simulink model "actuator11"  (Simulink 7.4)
settings: Solver=ode45  StartTime=0.0  StopTime=.35  MaxStep=1e-4  RelTol=1e-3
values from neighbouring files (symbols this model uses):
  D = str2num(get(h,'string'))    [acttrcalc1.m]
  fa = str2num(get(h,'string'))    [actsscalc1.m]    (also in acttrcalc1.m; calc0.m = f)
  k = str2num(get(h,'string'))    [actsscalc1.m]    (also in acttrcalc1.m; dcm.m = menu('DC MACHINES DEMOS:','DC motor transient running operat; dtcvectorselection.m = 1:6; dtcvectorsmovie.m = 1:6)
  K = 2.5    [actss.m]    (also in actsscalc1.m = str2num(get(h,'string')); acttrcalc1.m = str2num(get(h,'string')))
  M = length(wmm)    [Actac.m]    (also in acttrcalc1.m = str2num(get(h,'string')); calc0.m = fix(tf/ti))
  R = str2num(get(h,'string'))    [acttrcalc1.m]    (also in IMabc2.m = diag([Rs Rs Rs Rr Rr Rr]); IMabcf0.m = diag([Rs Rs Rs Rr Rr Rr]); IMabcf1.m = diag([Rs Rs Rs Rr Rr Rr]); IMcurf0.m = diag([Rs Rs Rr Rr]))
  V = [Vas 0 0].'    [Actac.m]    (also in acttrcalc1.m = str2num(get(h,'string')); im3d.m = eval(get(hVs,'String')); IMabc2.m = [vas vbs vcs 0 0 0]'; IMabcf0.m = [vas vbs vcs 0 0 0]')
  xsi = str2num(get(h,'string'))    [actsscalc1.m]    (also in acttrcalc1.m)

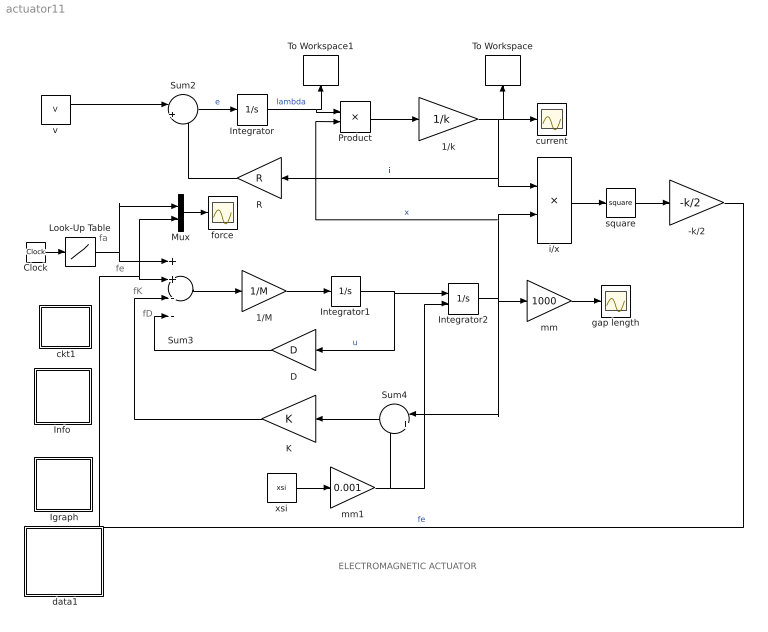
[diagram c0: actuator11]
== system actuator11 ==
  note: ELECTROMAGNETIC ACTUATOR
  note: fe
  note: fa
  note: fK
  note: fD
  " Igraph" : Subsystem
  " ckt1" : Subsystem
  " data1" : Subsystem
  -k/2 : Gain  Gain=-k/2  ParameterDataType=sfix(16)  ParameterScaling=2^0  OutDataType=sfix(16)  OutScaling=2^0
  1/M : Gain  Gain=1/M  ParameterDataType=sfix(16)  ParameterScaling=2^0  OutDataType=sfix(16)  OutScaling=2^0
  1/k : Gain  Gain=1/k  ParameterDataType=sfix(16)  ParameterScaling=2^0  OutDataType=sfix(16)  OutScaling=2^0
  Clock : Clock
  D : Gain  Gain=D  ParameterDataType=sfix(16)  ParameterScaling=2^0  OutDataType=sfix(16)  OutScaling=2^0
  Info : Subsystem
  Integrator : Integrator
  Integrator1 : Integrator
  Integrator2 : Integrator  InitialConditionSource=external  InitialCondition=0.003
  K : Gain  Gain=K  ParameterDataType=sfix(16)  ParameterScaling=2^0  OutDataType=sfix(16)  OutScaling=2^0
  Look-Up Table : Lookup  InputValues=[0 0.1 0.1 0.25 0.25 1]  Table=[0 0 fa fa 0 0]  OutDataType=sfix(16)  OutScaling=2^0
  Mux : Mux  Inputs=2
  Product : Product  OutDataType=sfix(16)  OutScaling=2^0
  R : Gain  Gain=R  ParameterDataType=sfix(16)  ParameterScaling=2^0  OutDataType=sfix(16)  OutScaling=2^0
  Sum2 : Sum  Inputs=|+-  OutDataType=sfix(16)  OutScaling=2^0
  Sum3 : Sum  Inputs=++--  OutDataType=sfix(16)  OutScaling=2^0
  Sum4 : Sum  Inputs=|+-  OutDataType=sfix(16)  OutScaling=2^0
  To Workspace : ToWorkspace  VariableName=i  SampleTime=-1  SaveFormat=Array
  To Workspace1 : ToWorkspace  VariableName=lambda  SampleTime=-1  SaveFormat=Array
  current : Scope
  force : Scope
  gap length : Scope
  i/x : Product  Inputs=*/  OutDataType=sfix(16)  OutScaling=2^0
  mm : Gain  Gain=1000  ParameterDataType=sfix(16)  ParameterScaling=2^0  OutDataType=sfix(16)  OutScaling=2^0
  mm1 : Gain  Gain=0.001  ParameterDataType=sfix(16)  ParameterScaling=2^0  OutDataType=sfix(16)  OutScaling=2^0
  square : Math  Operator=square
  v : Constant  Value=V  OutDataType=sfix(16)  OutScaling=2^0
  xsi : Constant  Value=xsi  OutDataType=sfix(16)  OutScaling=2^0
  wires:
  R/1 -> Sum2/2
  v/1 -> Sum2/1
  Sum2/1 -> Integrator/1  "e"
  Product/1 -> 1/k/1
  Sum3/1 -> 1/M/1
  D/1 -> Sum3/4
  K/1 -> Sum3/3
  square/1 -> -k/2/1
  1/k/1 -> i/x/1, R/1, current/1, To Workspace/1  "i"
  1/M/1 -> Integrator1/1
  i/x/1 -> square/1
  Sum4/1 -> K/1
  Mux/1 -> force/1
  -k/2/1 -> Sum3/2, Mux/2  "fe"
  Integrator/1 -> Product/1, To Workspace1/1  "lambda"
  Integrator1/1 -> D/1, Integrator2/1  "u"
  Look-Up Table/1 -> Sum3/1, Mux/1
  Clock/1 -> Look-Up Table/1
  Integrator2/1 -> Sum4/1, Product/2, i/x/2, mm/1  "x"
  mm/1 -> gap length/1
  xsi/1 -> mm1/1
  mm1/1 -> Integrator2/2, Sum4/2

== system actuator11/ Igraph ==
  note: This demo simulates the running of an induction motor
  note: Double click the block to enter the machine parameters and initial conditions and start the simulation

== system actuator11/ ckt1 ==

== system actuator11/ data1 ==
  note: This demo simulates the running of an induction motor in steady-state when a sudden input change is effected: a)torque step changes at constant voltage excitation b) voltage input sag at constant frequency and load torque c)simultaneous step changes in voltage magnitude and frequency
  note: Double click the block to enter the machine parameters and initial conditions and then run the simulation

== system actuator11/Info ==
  note: This demonstration illustrates the dynamic performance of an electromagnetic actuator modeled by a position-dependent inductance expressed by L(x) = k/x. Electrical system: v = Ri + d(lambda)/dt ; lambda = L(x) i or i = lambda* x / k Mechanical system: fa = Mdu/dt + Du + K(x-xsi) - fe ; fe = 0.5 i^2 dL/dx = -0.5*k*(i / x)^2 xsi = equilibrium position when i = 0 and fa = 0
  note: Electromagnetic actuator
  note: First enter the parameters by double clicking the corresponding block. Double click following the simulation.
